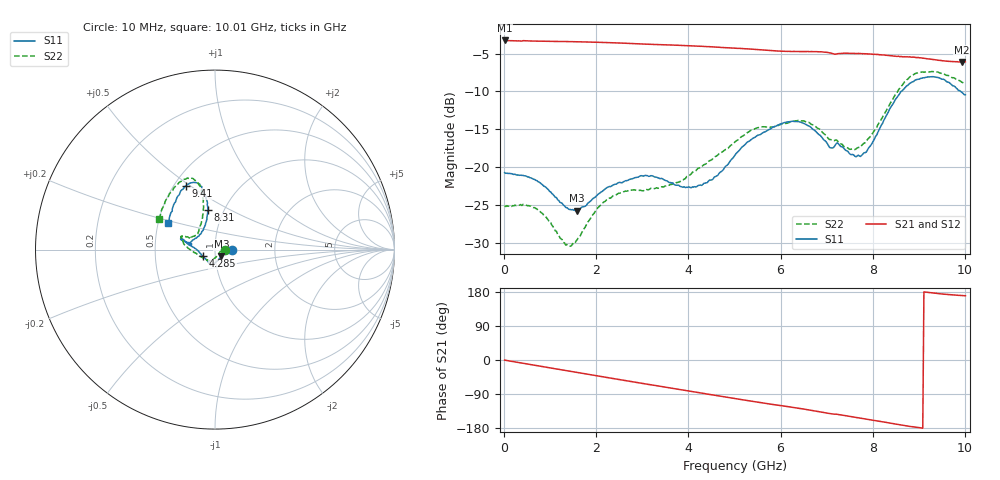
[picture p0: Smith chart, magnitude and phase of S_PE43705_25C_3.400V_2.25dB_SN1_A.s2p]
! Device ID: PE43705
! Serial: 1
! Insertion: A
! Impedance: 50 ohm
! Temp: 25C
! VDD: 3.400V
! Attenuation Step: 2.25dB
#  Hz  S  RI  R  50
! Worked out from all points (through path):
!   401 points, 10 MHz to 10.01 GHz, reference 50 ohm
!   highest |S21| = -3.27 dB at 10 MHz (marker M1); lowest = -6.1 dB at 9.935 GHz (marker M2)
!   group delay of S21, straight-line fit = 54.1 ps
!   lowest |S11| = -25.7 dB at 1.585 GHz (marker M3), VSWR 1.11, Z = 53.5 - j4.05 ohm
!   |S11| at or under -10 dB: start of sweep to 8.616 GHz; 9.908 GHz to end of sweep
!   |S22| runs from -30.4 to -7.4 dB; largest |S21 - S12| = 0.0059
!   S11 on the Smith chart (normalised r, x): 10 MHz: 1.20, -0.00; 4.285 GHz: 0.87, -0.07; 8.31 GHz: 0.84, +0.39; 9.41 GHz: 0.57, +0.48; 10.01 GHz: 0.56, +0.18
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1e7  0.092 -0.000595  0.6861 -0.00337  0.6866 -0.00324  0.0558 -0.000192
6.35e8  0.0826 0.0103  0.6616 -0.156  0.6615 -0.1558  0.0518 0.0155
1.335e9  0.0502 -0.0205  0.5975 -0.3137  0.5976 -0.3134  0.028 -0.0124
1.585e9  0.0353 -0.0378  0.5644 -0.3652  0.5646 -0.3651  0.0168 -0.0286
1.685e9  0.0298 -0.0456  0.5504 -0.3847  0.5504 -0.3846  0.0108 -0.0354
2.285e9  0.000224 -0.0746  0.4501 -0.487  0.4504 -0.4869  -0.0176 -0.06
3.36e9  -0.0294 -0.0794  0.2318 -0.6009  0.2326 -0.6003  -0.0458 -0.0568
4.285e9  -0.066 -0.0372  0.0293 -0.6275  0.0299 -0.6272  -0.0968 -0.0259
5.01e9  -0.1194 0.0128  -0.124 -0.5975  -0.1236 -0.5976  -0.1467 0.00598
5.435e9  -0.1534 0.0333  -0.2051 -0.5639  -0.2047 -0.5646  -0.175 0.0359
6.035e9  -0.1848 0.0601  -0.2986 -0.5004  -0.2966 -0.5009  -0.1837 0.0606
6.685e9  -0.1735 0.0464  -0.3965 -0.4217  -0.3966 -0.4211  -0.1757 0.0746
7.085e9  -0.1303 0.0315  -0.4451 -0.352  -0.4459 -0.3524  -0.1393 0.0616
7.26e9  -0.1358 0.0415  -0.4542 -0.3312  -0.4528 -0.3321  -0.1272 0.0709
7.685e9  -0.0864 0.0832  -0.4995 -0.2608  -0.4985 -0.2606  -0.0946 0.0962
7.91e9  -0.0628 0.1183  -0.5141 -0.2173  -0.5144 -0.2202  -0.083 0.1311
8.31e9  -0.0405 0.2198  -0.5289 -0.1411  -0.5273 -0.1438  -0.0644 0.2326
8.36e9  -0.0404 0.2365  -0.5296 -0.1305  -0.5284 -0.1327  -0.0647 0.2504
8.86e9  -0.0835 0.3561  -0.5312 -0.0364  -0.5284 -0.0394  -0.1134 0.3872
9.41e9  -0.1614 0.3559  -0.5073 0.0415  -0.506 0.0412  -0.1982 0.376
9.935e9  -0.2534 0.1812  -0.4873 0.0842  -0.4887 0.0845  -0.3011 0.2036
1.001e10  -0.2624 0.1475  -0.4882 0.0898  -0.4898 0.0886  -0.3133 0.1717
